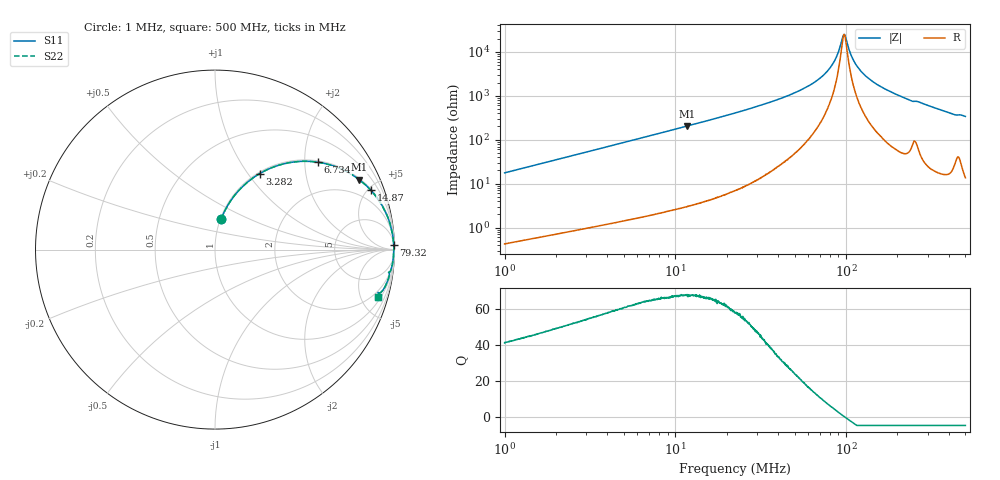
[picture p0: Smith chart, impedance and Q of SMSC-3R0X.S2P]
!s-Parameter Generated by FASTRON Sdn. Bhd.
!FASTRON P/N : SMSC-3R0X
!Keysight Technologies,E4991B,MY54100416,A.01.15
!Date: Mon Mar 16 10:11:59 2026
!Version  : Rev00 Mon Mar 16 10:11:59 2026
!Data & Calibration Information:
!PortZ  Port1:50+j0  Port2:50+j0
!When reading, reference impedance value at option line is always used.
! Remarks : This data is being provided solely for informational purposes.
!Freq	S11	S21	S12	S22
# Hz S dB R 50
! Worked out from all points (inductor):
!   1601 points, 1 MHz to 500 MHz, reference 50 ohm
!   read as one part in series: L = 2.79 uH near 1.032 MHz
!   highest Q = 68 at 11.78 MHz (marker M1), where L = 2.77 uH
!   self-resonance near 97.08 MHz
!   S11 on the Smith chart (normalised r, x): 1 MHz: 1.01, +0.35; 3.282 MHz: 1.02, +1.14; 6.734 MHz: 1.04, +2.33; 14.87 MHz: 1.08, +5.22; 79.32 MHz: 13, +79; 500 MHz: 1.27, -6.77
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1000000  -15.26 78.7  -0.17 -9.9  -0.17 -9.9  -15.26 78.7
1769978  -10.64 71.7  -0.45 -17.1  -0.45 -17.1  -10.64 71.7
2820919  -7.19 63.0  -1.00 -25.9  -1.00 -25.9  -7.19 63.0
3282298  -6.18 59.6  -1.29 -29.4  -1.29 -29.4  -6.18 59.6
6733586  -2.46 40.3  -3.79 -48.9  -3.79 -48.9  -2.46 40.3
7957584  -1.90 35.7  -4.69 -53.5  -4.69 -53.5  -1.90 35.7
1.178023e7  -0.98 25.8  -7.22 -63.3  -7.22 -63.3  -0.98 25.8
1.487185e7  -0.64 20.8  -8.97 -68.3  -8.97 -68.3  -0.64 20.8
2.236068e7  -0.29 13.8  -12.43 -75.2  -12.43 -75.2  -0.29 13.8
4.227946e7  -0.09 6.4  -19.11 -81.8  -19.11 -81.8  -0.09 6.4
6.307767e7  -0.04 3.1  -25.42 -83.0  -25.42 -83.0  -0.04 3.1
7.932318e7  -0.04 1.4  -32.05 -79.8  -32.05 -79.8  -0.04 1.4
8.673569e7  -0.03 0.8  -36.79 -73.8  -36.79 -73.8  -0.03 0.8
9.520996e7  -0.03 0.2  -46.30 -35.2  -46.30 -35.2  -0.03 0.2
9.783413e7  -0.03 -0.0  -47.89 7.0  -47.89 7.0  -0.03 -0.0
1.001409e8  -0.03 -0.2  -45.74 38.9  -45.74 38.9  -0.03 -0.2
1.090743e8  -0.04 -0.8  -37.06 72.4  -37.06 72.4  -0.04 -0.8
1.206648e8  -0.04 -1.5  -31.70 79.4  -31.70 79.4  -0.04 -1.5
1.420459e8  -0.05 -2.6  -26.69 82.0  -26.69 82.0  -0.05 -2.6
1.77937e8  -0.07 -4.4  -22.27 82.1  -22.27 82.1  -0.07 -4.4
2.399685e8  -0.16 -7.3  -17.87 78.1  -17.87 78.1  -0.16 -7.3
5e8  -0.46 -16.3  -11.05 71.4  -11.05 71.4  -0.46 -16.3
